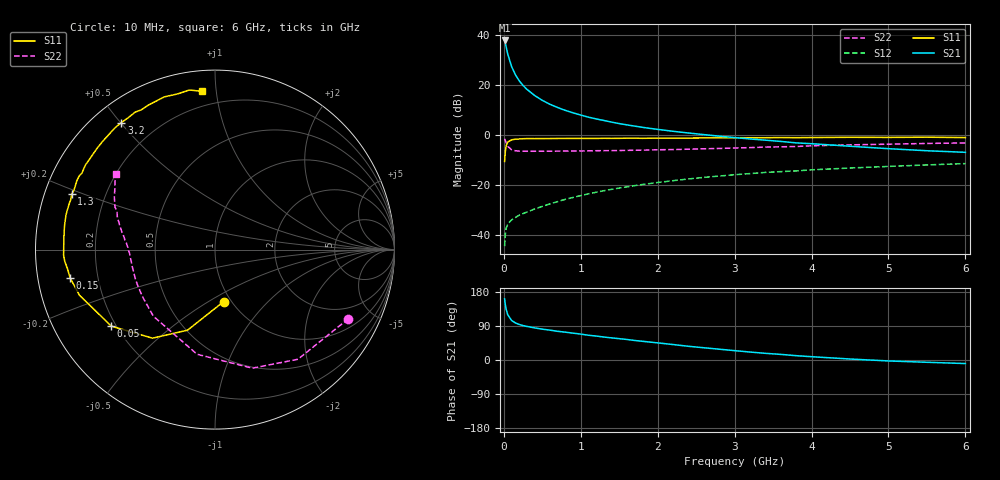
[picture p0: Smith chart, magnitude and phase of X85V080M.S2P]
! SIEMENS Small Signal Semiconductors
! BFP136W
! Si NPN RF Bipolar Junction Transistor in SOT343
! VCE = 5 V  IC = 80 mA
! Common Emitter S-Parameters:  September  1994
# GHz  S  MA  R  50
!  f  S11  S21  S12  S22
! GHz  MAG  ANG  MAG  ANG  MAG  ANG  MAG  ANG
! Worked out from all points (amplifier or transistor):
!   40 points, 10 MHz to 6 GHz, reference 50 ohm
!   highest |S21| = 37.9 dB at 10 MHz (marker M1)
!   |S21| within 3 dB of that: start of sweep to 33.25 MHz
!   unconditionally stable (mu >= 1): 613.5 MHz to 2.913 GHz
!   at 200 MHz: K = 0.62, MSG = 26.9 dB, |S12| = -32.1 dB
!   at 1.5 GHz: K = 1.10, MAG = 11.0 dB, |S12| = -21.3 dB
!   at 6 GHz: K = 0.97, MSG = 2.3 dB, |S12| = -11.5 dB
!   S11 on the Smith chart (normalised r, x): 10 MHz: 0.92, -0.59; 50 MHz: 0.18, -0.32; 150 MHz: 0.10, -0.10; 1.3 GHz: 0.08, +0.19; 3.2 GHz: 0.08, +0.50; 6 GHz: 0.11, +0.91
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0.01  0.294 -80.7  78.15 161.3  0.0059 69.9  0.8371 -27.4
0.02  0.4742 -108.8  68.02 145.6  0.0102 59.4  0.766 -52.9
0.03  0.6039 -125.2  58.3 134.1  0.0134 51.6  0.6926 -72.5
0.05  0.7183 -143.6  42.21 119.7  0.0163 40.1  0.5917 -99.7
0.1  0.7967 -161.4  23.59 104.5  0.0198 35.6  0.5057 -132.8
0.15  0.822 -168.8  16.12 97.9  0.0221 37.2  0.4816 -147.1
0.2  0.8289 -172.6  12.13 93.8  0.0247 38.6  0.4747 -155.1
0.25  0.84 -175.7  9.786 90.8  0.0265 41.4  0.4726 -160.0
0.3  0.8441 -177.9  8.19 88.6  0.0285 43.7  0.4703 -163.5
0.4  0.8431 178.2  6.171 84.7  0.0328 46.8  0.4705 -168.0
0.5  0.8444 175.3  4.926 81.4  0.037 50.2  0.471 -171.1
0.6  0.8463 173.2  4.108 78.8  0.0415 52.6  0.4717 -173.1
0.7  0.8492 170.6  3.541 75.7  0.0462 55.1  0.4738 -174.5
0.9  0.8524 166.9  2.771 70.8  0.0559 56.9  0.4761 -177.1
1.1  0.8515 162.4  2.266 65.3  0.066 57.8  0.48 -178.8
1.3  0.856 158.8  1.947 60.6  0.0763 58.4  0.4835 179.4
1.7  0.8608 151.6  1.502 51.5  0.0962 57.0  0.493 176.4
2.2  0.8618 143.4  1.182 40.8  0.1211 54.1  0.5088 172.8
3.2  0.8793 126.4  0.83 21.0  0.1679 45.4  0.5566 164.1
4.5  0.8965 108.4  0.593 2.6  0.2173 33.6  0.6323 152.5
5.5  0.9005 99.1  0.482 -6.0  0.2505 25.9  0.6752 145.6
6  0.8848 94.7  0.448 -9.4  0.2666 21.5  0.6916 142.6
